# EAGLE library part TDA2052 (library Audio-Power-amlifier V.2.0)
TDA2052 60W Hi-Fi AUDIO POWER AMPLIFIER WITH MUTE / STAND-BY
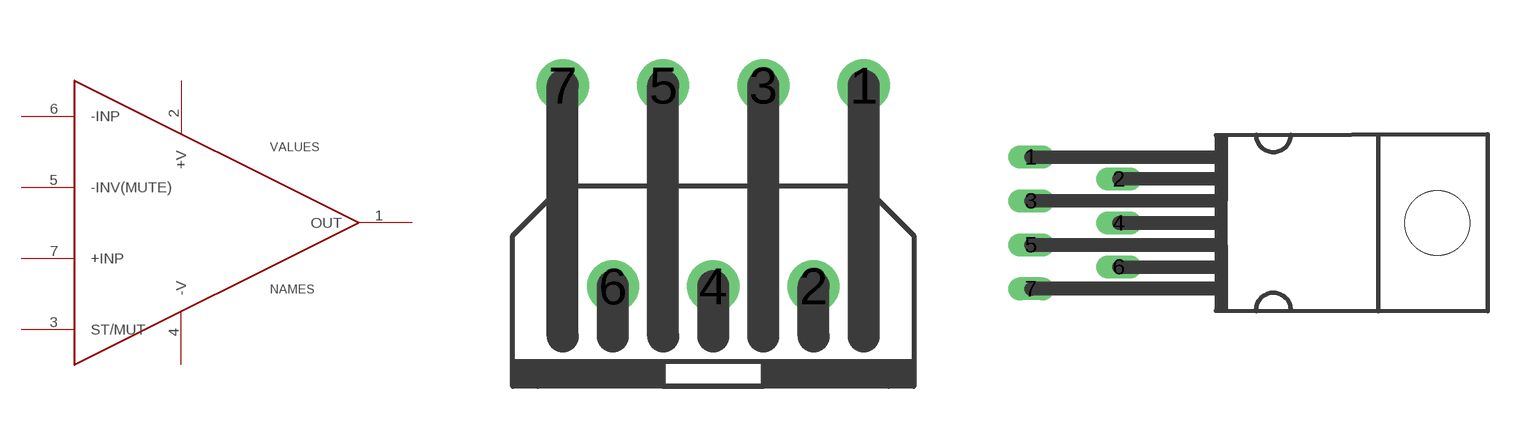
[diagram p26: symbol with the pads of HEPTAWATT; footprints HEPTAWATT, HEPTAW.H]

Designator prefix -

## TDA2052TDA2052V  [HEPTAWATT]
1  OUT  out
2  +V  pwr
3  ST/MUT
4  -V  pwr
5  -INV(MUTE)  in
6  -INP  in
7  +INP  in

## TDA2052TDA2052H  [HEPTAW.H]
Pads as for HEPTAWATT

## Footprint HEPTAWATT (pad centres in mm)
HEPTAWATT 7
drill 0.813: 1 3.81,5.08; 2 2.54,0; 3 1.27,5.08; 4 0,0; 5 -1.27,5.08; 6 -2.54,0; 7 -3.81,5.08

## Footprint HEPTAW.H (pad centres in mm)
drill 0.813 long: 1 -11.43,3.81; 2 -6.35,2.54; 3 -11.43,1.27; 4 -6.35,0; 5 -11.43,-1.27; 6 -6.35,-2.54; 7 -11.43,-3.81
hole 3.75 at 12.05,0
